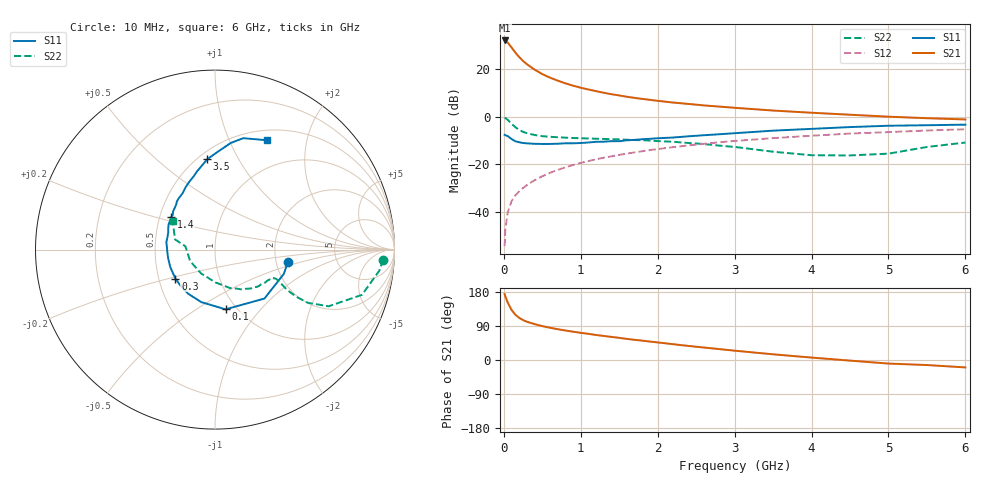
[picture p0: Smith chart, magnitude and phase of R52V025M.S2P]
! SIEMENS Small Signal Semiconductors
! BFR183
! Si NPN RF Bipolar Junction Transistor in SOT23
! VCE = 2 V  IC = 25 mA
! Common Emitter S-Parameters:  May  1996
# GHz  S  MA  R  50
!  f  S11  S21  S12  S22
! GHz  MAG  ANG  MAG  ANG  MAG  ANG  MAG  ANG
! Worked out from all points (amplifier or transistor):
!   36 points, 10 MHz to 6 GHz, reference 50 ohm
!   highest |S21| = 31.9 dB at 10 MHz (marker M1)
!   |S21| within 3 dB of that: start of sweep to 101.2 MHz
!   unconditionally stable (mu >= 1): 435.5 MHz to 2.386 GHz
!   at 250 MHz: K = 0.88, MSG = 26.7 dB, |S12| = -30.0 dB
!   at 1.4 GHz: K = 1.06, MAG = 11.6 dB, |S12| = -16.7 dB
!   at 6 GHz: K = 0.91, MSG = 2.1 dB, |S12| = -5.3 dB
!   S11 on the Smith chart (normalised r, x): 10 MHz: 2.32, -0.40; 100 MHz: 0.89, -0.67; 300 MHz: 0.61, -0.21; 1.4 GHz: 0.57, +0.23; 3.5 GHz: 0.55, +0.75; 6 GHz: 0.62, +1.39
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0.01  0.412 -10.0  39.49 173.8  0.0019 91.6  0.9396 -3.4
0.02  0.4066 -19.5  39.01 167.7  0.0043 85.6  0.9231 -7.3
0.05  0.3876 -44.7  35.72 151.8  0.0097 75.3  0.857 -17.1
0.1  0.3379 -80.0  28.12 132.2  0.0167 70.8  0.7076 -26.5
0.15  0.3023 -104.6  21.95 119.3  0.0221 68.0  0.5964 -29.8
0.2  0.2879 -121.3  17.71 111.2  0.0269 69.3  0.5243 -30.1
0.25  0.278 -133.9  14.66 105.3  0.0316 69.5  0.4762 -29.5
0.3  0.2733 -143.9  12.52 100.9  0.0364 70.5  0.4469 -28.7
0.4  0.2675 -158.6  9.637 94.7  0.046 72.1  0.4095 -27.0
0.5  0.2655 -169.2  7.769 89.4  0.0557 72.7  0.3868 -25.9
0.6  0.2658 -176.6  6.556 85.1  0.0657 72.5  0.3753 -25.6
0.7  0.2685 176.8  5.669 81.3  0.0757 72.7  0.3675 -25.8
0.8  0.274 171.6  4.974 77.9  0.0857 71.7  0.3601 -26.1
0.9  0.2739 165.3  4.438 74.7  0.0962 71.3  0.3535 -26.5
1.1  0.2854 156.1  3.69 69.0  0.1163 70.1  0.346 -28.9
1.4  0.3041 143.5  2.937 60.9  0.146 67.2  0.3358 -32.7
1.7  0.3236 133.7  2.46 53.2  0.1766 64.1  0.3209 -37.4
2.2  0.3621 119.9  1.964 41.7  0.2273 58.3  0.295 -47.3
3.5  0.5054 94.9  1.335 15.0  0.3517 41.2  0.1825 -89.4
4.5  0.6004 81.6  1.091 -1.6  0.4392 28.0  0.1526 -155.1
5.5  0.6563 69.4  0.922 -13.3  0.5091 16.0  0.2295 165.7
6  0.6751 64.5  0.868 -19.6  0.5409 8.3  0.2842 146.1
